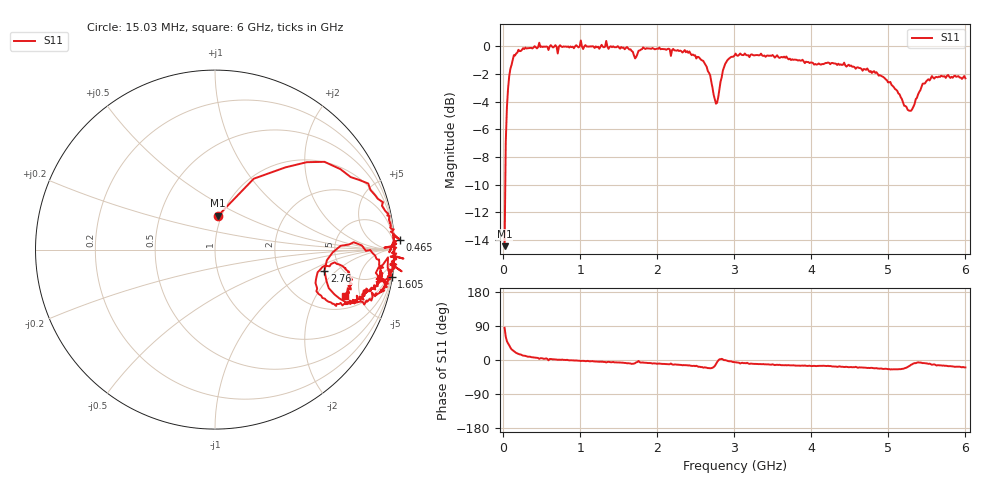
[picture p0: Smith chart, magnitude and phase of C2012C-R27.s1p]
!	Network	Analyzer	HP8753E.07.74:	Oct	30	2002	Serial	No.	JP38451487
!	Hewlett-Packard
!	7	Sep	2009	12:22:38
!	Frequency	S11
#	HZ	S	RI	R	50
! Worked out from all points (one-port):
!   400 points, 15.03 MHz to 6 GHz, reference 50 ohm
!   lowest |S11| = -14.4 dB at 15.03 MHz (marker M1), VSWR 1.47, Z = 48.1 + j18.9 ohm
!   |S11| at or under -10 dB: start of sweep to 23.9 MHz
!   S11 on the Smith chart (normalised r, x): 15.03 MHz: 0.96, +0.38; 465 MHz: -17, +28; 1.605 GHz: 0, -13; 2.76 GHz: 3.70, -1.42; 6 GHz: 2.89, -3.60
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1.502992e7  0.0172 0.189
3.002985e7  0.216 0.395
4.502978e7  0.392 0.458
9.002955e7  0.699 0.448
1.350293e8  0.854 0.368
4.650277e8  1.03 0.0543
7.650262e8  0.995 0.0205
1.005025e9  1.05 -0.0501
1.035025e9  0.978 -0.0388
1.335023e9  1.04 -0.121
1.515022e9  0.975 -0.114
1.605022e9  0.984 -0.152
1.710021e9  0.896 -0.13
1.755021e9  0.964 -0.0434
1.785021e9  0.967 -0.12
2.265019e9  0.948 -0.207
2.535017e9  0.871 -0.284
2.685017e9  0.73 -0.293
2.760016e9  0.61 -0.118
2.835016e9  0.773 0.041
3.015015e9  0.937 -0.1
3.765011e9  0.868 -0.216
4.515007e9  0.809 -0.272
5.025005e9  0.675 -0.314
5.265004e9  0.562 -0.169
5.385003e9  0.667 -0.071
5.565002e9  0.763 -0.169
6e9  0.723 -0.256
